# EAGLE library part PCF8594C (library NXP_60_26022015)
The PCF8594C-2 is a ?oating gate Electrically Erasable Programmable Read Only Memory (EEPROM) with 4 kbits (512 × 8-bit) non-volatile storage. AAL Eindhoven MK
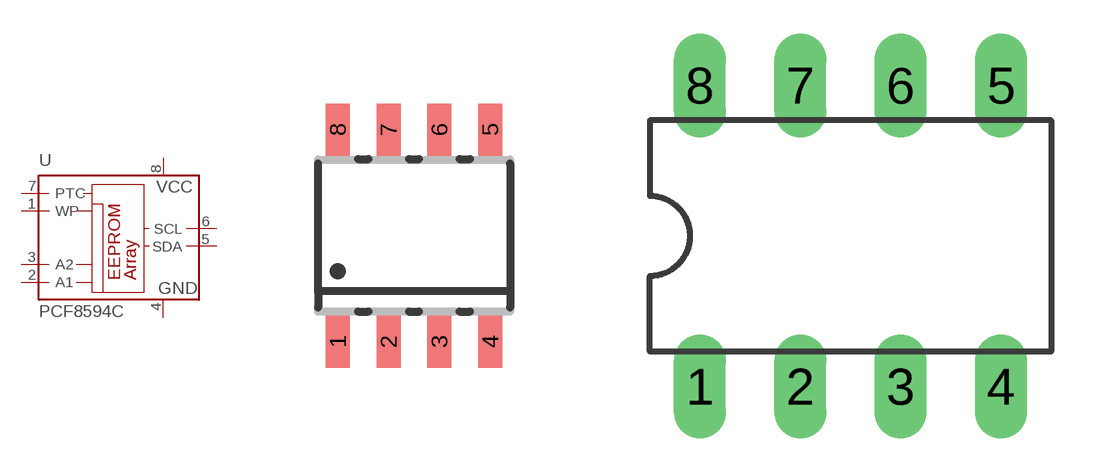
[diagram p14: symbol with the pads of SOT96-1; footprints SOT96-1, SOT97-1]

Designator prefix U

## PCF8594CC-2T/02 (SAMPLEDESK: 12NC935195550118)  [SOT96-1]
1  WP  in
2  A1  in
3  A2  in
4  GND  pwr
5  SDA
6  SCL  in
7  PTC
8  VCC  pwr

## PCF8594CC-2P/02  [SOT97-1]
Pads as for SOT96-1

## Footprint SOT96-1 (pad centres in mm)
SOT96-1 SO8: plastic small outline package; 8 leads; body width 3.9 mm JEDEC: MS-012 IEC: 076E03
smd 0.6 x 1.3: 1 -1.905,-2.65; 2 -0.635,-2.65; 3 0.635,-2.65; 4 1.905,-2.65; 5 1.905,2.65; 6 0.635,2.65; 7 -0.635,2.65; 8 -1.905,2.65

## Footprint SOT97-1 (pad centres in mm)
Dual In Line Package
drill 0.813 long: 1 -3.81,-3.81; 2 -1.27,-3.81; 3 1.27,-3.81; 4 3.81,-3.81; 5 3.81,3.81; 6 1.27,3.81; 7 -1.27,3.81; 8 -3.81,3.81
